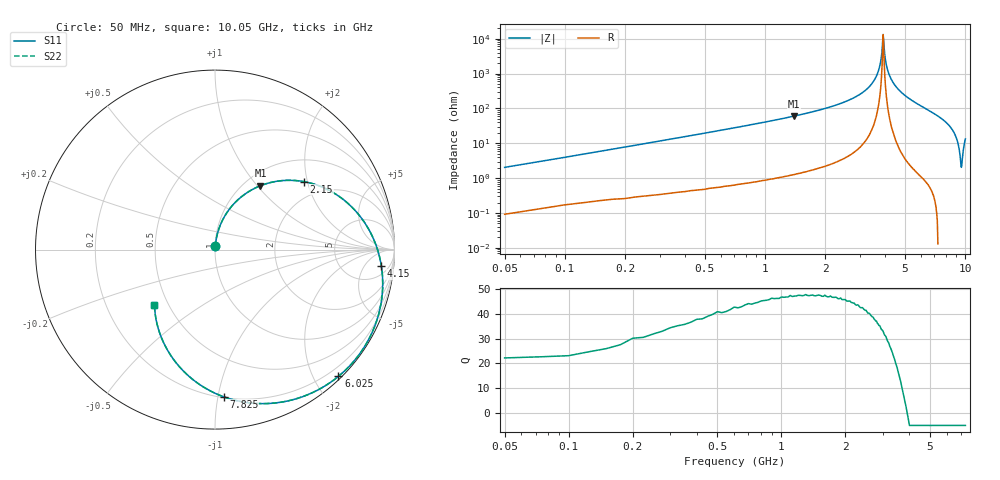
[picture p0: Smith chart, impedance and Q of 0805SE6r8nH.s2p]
! AVX Thin Film Operation		Date: May 2002
! Description: Accu-L® Series, Thin Film, SMD, RF Inductors
! Part Number: L08056R8CEWTR
! 50 MHz  -  10.05 GHz
! Serial Measurements
# mhz S db R 50
!	S11		S21		S12		S22
!	dB	Phase	dB	Phase	dB	Phase	dB	Phase
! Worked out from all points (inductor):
!   401 points, 50 MHz to 10.05 GHz, reference 50 ohm
!   read as 1/Y11, port 2 shorted: L = 6.25 nH near 100 MHz
!   highest Q = 47.4 at 1.4 GHz (marker M1), where L = 6.86 nH
!   self-resonance near 3.9 GHz
!   S11 on the Smith chart (normalised r, x): 50 MHz: 1.00, +0.04; 2.15 GHz: 1.54, +1.90; 4.15 GHz: 10, -13; 6.025 GHz: 0.05, -2.37; 7.825 GHz: 0.21, -1.04; 10.05 GHz: 0.42, -0.33
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50  -34.91 85.5  -0.01 -1.3  -0.01 -1.3  -34.91 85.5
200  -23.34 82.8  -0.04 -5.0  -0.04 -5.0  -23.34 82.8
450  -16.48 77.1  -0.14 -11.1  -0.14 -11.1  -16.48 77.1
850  -11.17 67.6  -0.40 -20.8  -0.40 -20.8  -11.17 67.6
1400  -7.20 54.6  -0.99 -33.7  -0.99 -33.7  -7.20 54.6
1725  -5.64 47.0  -1.47 -41.2  -1.47 -41.2  -5.64 47.0
2150  -4.10 37.4  -2.25 -50.7  -2.25 -50.7  -4.10 37.4
3400  -1.44 10.1  -5.73 -77.2  -5.73 -77.2  -1.44 10.1
4150  -0.61 -5.7  -9.25 -92.4  -9.25 -92.4  -0.61 -5.7
4675  -0.27 -16.7  -13.22 -102.6  -13.22 -102.6  -0.27 -16.7
5050  -0.12 -24.7  -18.03 -109.2  -18.03 -109.2  -0.12 -24.7
5325  -0.07 -30.6  -24.95 -111.5  -24.95 -111.5  -0.07 -30.6
5400  -0.06 -32.2  -28.46 -110.5  -28.46 -110.5  -0.06 -32.2
5500  -0.06 -34.3  -37.56 -95.8  -37.56 -95.8  -0.06 -34.3
5550  -0.06 -35.4  -37.13 -31.0  -37.13 -31.0  -0.06 -35.4
5775  -0.07 -40.3  -24.69 47.2  -24.69 47.2  -0.07 -40.3
6025  -0.12 -45.8  -18.28 45.0  -18.28 45.0  -0.12 -45.8
6725  -0.48 -61.4  -10.50 31.5  -10.50 31.5  -0.48 -61.4
7825  -1.71 -86.7  -5.14 7.8  -5.14 7.8  -1.71 -86.7
8400  -2.71 -100.0  -3.54 -4.8  -3.54 -4.8  -2.71 -100.0
9200  -4.50 -118.4  -2.08 -21.9  -2.08 -21.9  -4.50 -118.4
10050  -6.81 -137.7  -1.17 -39.4  -1.17 -39.4  -6.81 -137.7
